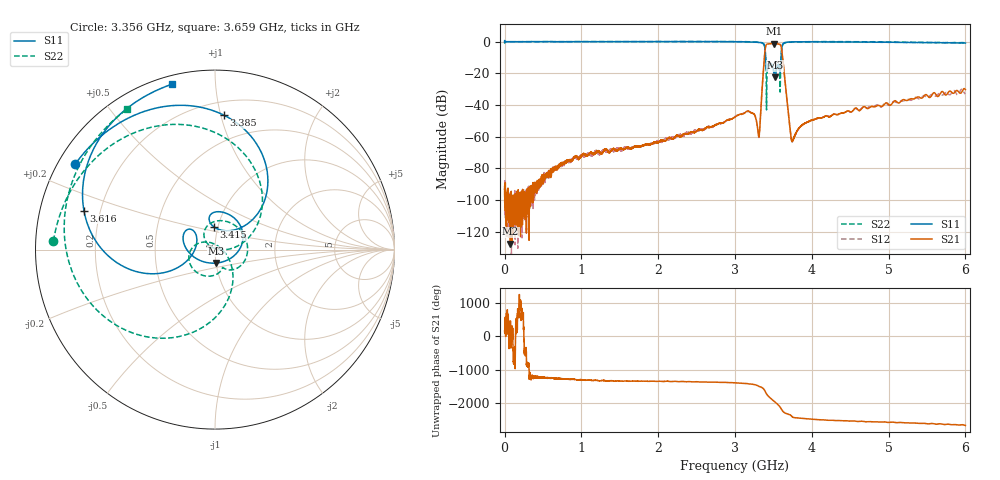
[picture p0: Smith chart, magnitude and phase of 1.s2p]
#  HZ  S  MA  R  50.00
! Rohde & Schwarz Vector Network Analyzer
! Rohde-Schwarz,ZNL6-2Port,1323001206101378,1.50.1.34-21.10.1.104
! Created: UTC 8/22/2024, 7:47:22 AM
! freq[Hz]  mag:S11  ang:S11  mag:S21  ang:S21  mag:S12  ang:S12  mag:S22  ang:S22
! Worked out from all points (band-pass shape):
!   10001 points, 5 kHz to 6 GHz, reference 50 ohm
!   highest |S21| = -1.14 dB at 3.511 GHz (marker M1); lowest = -127.6 dB at 75 MHz (marker M2)
!   |S21| within 3 dB of the highest: 3.395 GHz to 3.605 GHz (210.2 MHz wide, 6.01 % of centre)
!   lowest |S11| = -22.5 dB at 3.519 GHz (marker M3), VSWR 1.16, Z = 50.1 - j7.56 ohm
!   |S11| at or under -10 dB: 3.4 GHz to 3.599 GHz (198.9 MHz wide, 5.68 % of centre)
!   |S22| runs from -43.1 to 0.1 dB; largest |S21 - S12| = 0.017
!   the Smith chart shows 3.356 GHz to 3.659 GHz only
!   S11 on the Smith chart (normalised r, x): 3.356 GHz: 0.05, +0.28; 3.385 GHz: 0.30, +1.02; 3.415 GHz: 0.96, +0.25; 3.616 GHz: 0.14, +0.14; 3.659 GHz: 0.04, +0.77
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5000  0.9995 0.2  2.183e-05 160.9  2.338e-05 -56.9  0.9969 0.2
7.500494e7  1.001 -0.5  4.153e-07 -105.1  9.013e-06 52.1  0.9986 -1.0
1.000204e9  1.002 -8.6  0.0002497 148.2  0.0002591 144.1  1.001 -9.6
2.000403e9  1.01 -22.2  0.0006467 98.5  0.0007533 97.1  1.004 -23.4
3.000002e9  1.001 -61.8  0.00418 54.8  0.004269 56.6  0.9993 -57.1
3.204602e9  0.9729 -102.5  0.005794 14.6  0.005868 15.1  0.9849 -88.0
3.303602e9  0.9464 -154.5  0.001206 -39.9  0.00119 -39.6  0.959 -128.6
3.327602e9  0.9411 -175.9  0.002941 -66.4  0.002872 -65.8  0.9503 -147.7
3.356402e9  0.913 148.6  0.04249 -96.5  0.0435 -96.4  0.9013 177.0
3.384602e9  0.7503 86.2  0.3628 -167.4  0.3566 -167.9  0.7065 101.5
3.415202e9  0.126 92.4  0.8355 65.7  0.832 66.3  0.07267 137.1
3.451802e9  0.2125 75.7  0.8615 -25.2  0.8626 -24.6  0.181 18.5
3.481202e9  0.1833 33.4  0.8725 -83.6  0.8765 -83.0  0.1582 -42.4
3.510602e9  0.08947 -41.6  0.8767 -138.8  0.8762 -138.4  0.1093 -66.2
3.519002e9  0.07532 -84.8  0.8755 -154.8  0.8762 -154.3  0.1097 -68.0
3.565802e9  0.1954 150.0  0.8423 107.8  0.8373 108.4  0.1601 -150.2
3.616202e9  0.7619 163.4  0.3798 -55.7  0.389 -55.6  0.7221 -148.9
3.659402e9  0.9519 104.6  0.03564 -136.2  0.03521 -136.2  0.9236 121.9
3.748802e9  0.9855 62.1  0.0007488 116.5  0.0007385 114.4  0.9752 61.9
4.000202e9  1 22.4  0.003323 49.0  0.00332 48.9  1.002 15.0
5.000401e9  0.9517 -7.2  0.01034 -48.3  0.009777 -45.5  0.9824 -11.8
6e9  0.9071 -22.7  0.03077 -138.4  0.02224 -129.2  0.9163 -25.9
